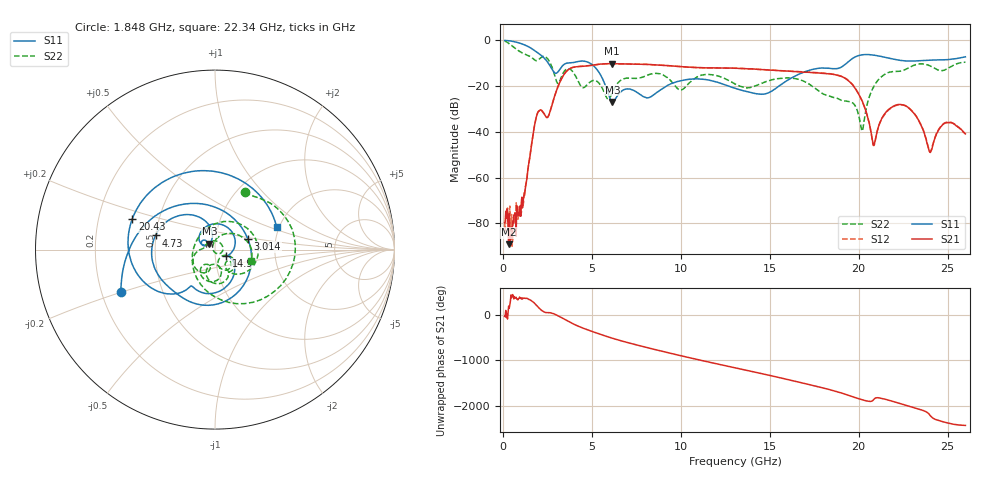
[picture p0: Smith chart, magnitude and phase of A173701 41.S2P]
!  2-Port S-parameters saved by WinCal
! VAR MeasName=S-Parameters (CALIBRATED_DATA) read from VNA (N5245A)
! VAR MeasDate=2017-6-7 10:31:09
! VAR NAME=A173701 41
! VAR FILENAME=A173701 41.S2P
! VAR DATE=2017-6-7 10:31:09
! VAR PHYS_PORTS=1,2
# Hz S DB R 50
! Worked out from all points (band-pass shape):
!   801 points, 100 MHz to 26 GHz, reference 50 ohm
!   highest |S21| = -10.15 dB at 6.122 GHz (marker M1); lowest = -89.0 dB at 326.6 MHz (marker M2)
!   |S21| within 3 dB of the highest: 3.623 GHz to 15.45 GHz (11.82 GHz wide, 124 % of centre)
!   lowest |S11| = -26.8 dB at 6.154 GHz (marker M3), VSWR 1.10, Z = 46.9 + j3.15 ohm
!   |S11| at or under -10 dB: 2.563 GHz to 3.571 GHz (1.008 GHz wide, 32.9 % of centre); 4.909 GHz to 19.31 GHz (14.4 GHz wide, 119 % of centre)
!   |S22| runs from -39.6 to -0.2 dB; largest |S21 - S12| = 0.0044
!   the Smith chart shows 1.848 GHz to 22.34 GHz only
!   S11 on the Smith chart (normalised r, x): 1.848 GHz: 0.28, -0.20; 3.014 GHz: 1.44, +0.18; 4.73 GHz: 0.50, +0.09; 14.9 GHz: 1.13, -0.08; 20.43 GHz: 0.35, +0.16; 22.34 GHz: 1.93, +0.57
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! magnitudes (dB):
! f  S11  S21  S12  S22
! 100 MHz  0.0  -79.7  -79.3  -0.2
! 326.6 MHz  -0.1  -89.0  -77.9  -1.3
! 1.104 GHz  -1.6  -73.2  -71.4  -5.5
! 1.848 GHz  -4.8  -34.7  -34.6  -8.8
! 3.014 GHz  -14.3  -22.0  -22.0  -17.8
! 4.438 GHz  -9.0  -11.3  -11.3  -20.5
! 4.73 GHz  -9.4  -11.1  -11.1  -19.4
! 6.122 GHz  -26.7  -10.1  -10.2  -23.3
! 6.154 GHz  -26.8  -10.2  -10.2  -22.7
! 8.744 GHz  -22.3  -10.7  -10.8  -14.5
! 13.05 GHz  -20.9  -12.2  -12.2  -19.0
! 14.9 GHz  -23.0  -12.9  -12.9  -17.7
! 17.39 GHz  -12.7  -14.1  -13.9  -20.0
! 19.36 GHz  -9.7  -17.2  -17.1  -26.6
! 20.17 GHz  -6.3  -26.1  -26.1  -39.4
! 20.43 GHz  -6.2  -31.5  -31.5  -29.5
! 20.85 GHz  -6.4  -45.9  -45.9  -20.2
! 21.69 GHz  -7.7  -30.1  -30.3  -14.0
! 22.34 GHz  -8.7  -28.0  -28.1  -13.4
! 23.99 GHz  -8.6  -48.7  -48.5  -11.0
! 24.87 GHz  -8.4  -36.1  -36.0  -12.8
! 26 GHz  -7.2  -40.9  -40.8  -9.5
